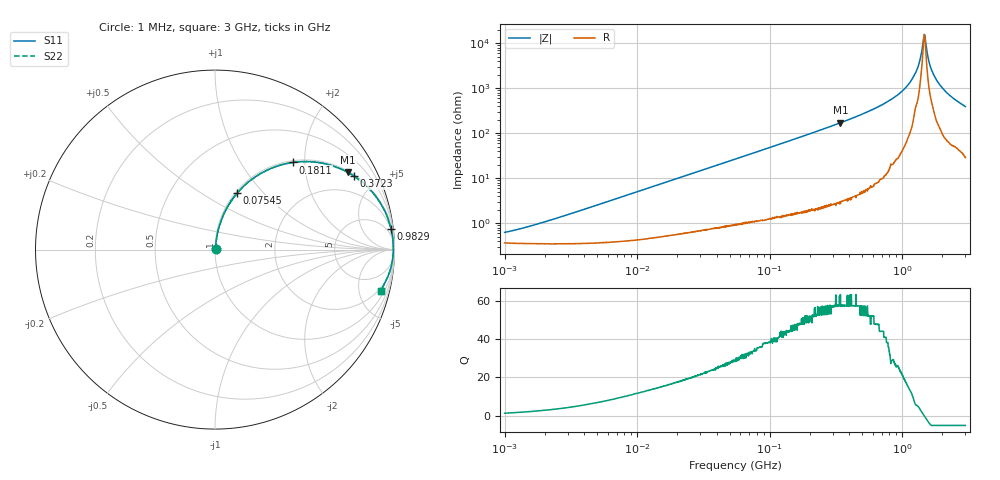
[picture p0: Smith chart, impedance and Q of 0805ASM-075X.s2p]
!s-Parameter Generated by FASTRON Sdn. Bhd.
!FASTRON P/N : 0805ASM-075X
!Keysight Technologies: E4991B_MY54100416_A.01.15
!Date: Fri Jun 19 14:49:41 2026
!Version  :Rev00  Fri Jun 19 14:49:41 2026
!Data & Calibration Information:
!Freq  S11  S21  S12  S22
!PortZ  Port1:50+j0  Port2:50+j0
!When reading reference impedance value at option line is always used.
! Remarks : This data is being provided solely for informational purposes.
# Hz S dB R 50
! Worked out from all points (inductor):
!   1601 points, 1 MHz to 3 GHz, reference 50 ohm
!   read as one part in series: L = 80.2 nH near 2.066 MHz
!   highest Q = 57.7 at 341.9 MHz (marker M1), where L = 79.6 nH
!   self-resonance near 1.467 GHz
!   S11 on the Smith chart (normalised r, x): 1 MHz: 1.01, +0.01; 75.45 MHz: 1.02, +0.73; 181.1 MHz: 1.04, +1.75; 372.3 MHz: 1.06, +3.76; 982.9 MHz: 2, +17; 3 GHz: 1.56, -7.78
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1000000  -44.10 53.9  -0.03 -0.3  -0.03 -0.3  -44.10 53.9
3804036  -34.30 78.5  -0.03 -1.1  -0.03 -1.1  -34.30 78.5
1.447069e7  -22.90 82.0  -0.06 -4.1  -0.06 -4.1  -22.90 82.0
5.504702e7  -11.90 73.2  -0.37 -14.8  -0.37 -14.8  -11.90 73.2
7.544761e7  -9.40 68.5  -0.62 -19.8  -0.62 -19.8  -9.40 68.5
1.811155e8  -3.71 48.1  -2.56 -40.7  -2.56 -40.7  -3.71 48.1
2.083556e8  -3.05 44.1  -3.14 -44.7  -3.14 -44.7  -3.05 44.1
3.419417e8  -1.34 30.1  -6.00 -59.0  -6.00 -59.0  -1.34 30.1
3.72303e8  -1.14 27.8  -6.63 -61.2  -6.63 -61.2  -1.14 27.8
7.925923e8  -0.20 10.7  -14.60 -77.7  -14.60 -77.7  -0.20 10.7
9.828732e8  -0.11 6.8  -18.50 -80.6  -18.50 -80.6  -0.11 6.8
1.130699e9  -0.07 4.4  -22.30 -81.5  -22.30 -81.5  -0.07 4.4
1.268618e9  -0.07 2.5  -27.20 -77.6  -27.20 -77.6  -0.07 2.5
1.347129e9  -0.06 1.5  -31.50 -74.8  -31.50 -74.8  -0.06 1.5
1.437675e9  -0.06 0.4  -40.50 -46.5  -40.50 -46.5  -0.06 0.4
1.474099e9  -0.05 -0.0  -44.00 5.4  -44.00 5.4  -0.05 -0.0
1.511446e9  -0.06 -0.5  -39.70 52.0  -39.70 52.0  -0.06 -0.5
1.581072e9  -0.06 -1.3  -32.80 72.1  -32.80 72.1  -0.06 -1.3
1.645649e9  -0.07 -2.0  -29.10 76.0  -29.10 76.0  -0.07 -2.0
1.855641e9  -0.09 -4.1  -22.90 79.2  -22.90 79.2  -0.09 -4.1
2.266846e9  -0.19 -7.9  -17.20 77.2  -17.20 77.2  -0.19 -7.9
3e9  -0.42 -14.1  -12.30 71.7  -12.30 71.7  -0.42 -14.1
